(* Logix 5000 AddOnInstructionDefinition export EGU_EGK_IO_Link_Cyclic_Com_1_0_1; software revision 35.00 *)

TYPE PROCESS_DATA_IN :
STRUCT
   B0_00 : BOOL;
   B0_01 : BOOL;
   B0_02 : BOOL;
   B0_03 : BOOL;
   B0_04 : BOOL;
   B0_05 : BOOL;
   B0_06 : BOOL;
   B0_07 : BOOL;
   B0_08 : BOOL;
   B0_09 : BOOL;
   B0_10 : BOOL;
   B0_11 : BOOL;
   B0_12 : BOOL;
   B0_13 : BOOL;
   B0_14 : BOOL;
   B0_15 : BOOL;
   B0_16 : BOOL;
   B0_17 : BOOL;
   B0_18 : BOOL;
   B0_19 : BOOL;
   B0_20 : BOOL;
   B0_21 : BOOL;
   B0_22 : BOOL;
   B0_23 : BOOL;
   B0_24 : BOOL;
   B0_25 : BOOL;
   B0_26 : BOOL;
   B0_27 : BOOL;
   B0_28 : BOOL;
   B0_29 : BOOL;
   B0_30 : BOOL;
   B0_31 : BOOL;
   DINT_1 : DINT;
   DINT_2 : DINT;
   SINT_3_0 : SINT;
   SINT_3_1 : SINT;
   SINT_3_2 : SINT;
   SINT_3_3 : SINT;
END_STRUCT
END_TYPE

TYPE PROCESS_DATA_OUT :
STRUCT
   DINT_0 : DINT;
   DINT_1 : DINT;
   DINT_2 : DINT;
   DINT_3 : DINT;
END_STRUCT
END_TYPE

ADD_ON_INSTRUCTION EGU_EGK_IO_Link_Cyclic_Com_1_0_1   (* revision 1.0 1, ExecutePrescan, ExecuteEnableInFalse *)
// FUNCTION_BLOCK FB_SFP_EGU/EGK Allen Breadley
// TITLE = 'EGU_EGK_Cyclic_Communication'
// VERSION : '1.0.1'
// AUTHOR  : 'SCHUNK'
// NAME    : 'EGU_EGK_Cyclic_Communication'
// FAMILY  : 'SCHUNK'
// Used Products : EGU / EGK
// Projekt Nr.:
// =============================================================================
//  Schunk GmbH&Co.KG
//  (c)Copyright (2022) All Rights Reserved
// -----------------------------------------------------------------------------
//  Library:       Schunk
//  Tested with:   V35.00.00
VAR_INPUT
   b_in_RELEASE_FUNCTION_BLOCK : BOOL; {access Read Only, visible}
   b_in_00_FAST_STOP : BOOL; {access Read Only, visible}
   b_in_01_STOP : BOOL; {access Read Only, visible}
   b_in_02_ACKNOLEDGE : BOOL; {access Read Only, visible}
   b_in_03_PREPARE_FOR_SHUTDOWN : BOOL; {access Read Only, visible}
   b_in_04_SOFTRESET : BOOL; {access Read Only, visible}
   b_in_05_RELEASE_FOR_MANUAL_MOVEMENT : BOOL; {access Read Only, visible}
   b_in_06_REPEAT_COMMAND_TOGGLE : BOOL; {access Read Only, visible}
   b_in_07_GRIP_DIRECTION : BOOL; {access Read Only, visible}
   b_in_08_JOG_MODE_NEGATIVE : BOOL; {access Read Only, visible}
   b_in_09_JOG_MODE_POSITIVE : BOOL; {access Read Only, visible}
   b_in_11_RELEASE_WORKPIECE : BOOL; {access Read Only, visible}
   b_in_12_GRIP_WORKPIECE : BOOL; {access Read Only, visible}
   b_in_13_MOVE_TO_ABSOLUTE_POSITION : BOOL; {access Read Only, visible}
   b_in_14_MOVE_TO_RELATIVE_POSITION : BOOL; {access Read Only, visible}
   b_in_16_GRIP_WORKPIECE_AT_EXPECTED_POS : BOOL; {access Read Only, visible}
   b_in_30_BRAKE_TEST : BOOL; {access Read Only, visible}
   b_in_31_ACTIVATE_GRIP_FORCE_AND_POS_MA : BOOL; {access Read Only, visible}
   di_in_POSITION : DINT; {access Read Only, visible}
   di_in_VELOCITY : DINT; {access Read Only, visible}
   di_in_GRIPPING_FORCE : DINT; {access Read Only, visible}
END_VAR
VAR_OUTPUT
   b_out_00_READY_FOR_OPERATION : BOOL; {visible}
   b_out_01_CONTOL_AUTHORITY_FIELDBUS : BOOL; {visible}
   b_out_02_READY_FOR_SHUTDOWN : BOOL; {visible}
   b_out_03_NOT_FEASIBLE : BOOL; {visible}
   b_out_04_COMMAND_SUCCESSFULLY_PROCESSED : BOOL; {visible}
   b_out_05_COMMAND_RECEIVED_TOGGLE : BOOL; {visible}
   b_out_06_WARNING : BOOL; {visible}
   b_out_07_ERROR : BOOL; {visible}
   b_out_08_RELEASED_FOR_MANUAL_MOVEMENT : BOOL; {visible}
   b_out_09_SOFTWARE_LIMIT_REACHED : BOOL; {visible}
   b_out_11_NO_WORKPIECE_DETECTED : BOOL; {visible}
   b_out_12_WORKPIECE_GRIPPED : BOOL; {visible}
   b_out_13_POSITION_REACHED : BOOL; {visible}
   b_out_14_WORKPIECE_PRE_GRIP_STARTED : BOOL; {visible}
   b_out_16_WORKPIECE_LOST : BOOL; {visible}
   b_out_17_WRONG_WORKPIECE_DETECTED : BOOL; {visible}
   b_out_31_GRIP_FORCE_AND_POS_MAINTAINANC : BOOL; {visible}
   di_out_ACTUAL_POSITION : DINT; {visible}
   si_out_DIAGNOSIS_ERROR : SINT; {visible}
   si_out_DIAGNOSIS_WARNING : SINT; {visible}
   si_out_DIAGNOSIS_WARNING_CODE : SINT;
END_VAR
VAR_INPUT
   in_PROCESS_DATA_INPUT : DINT; {access Read Only}
END_VAR
VAR_IN_OUT
   in_PROZESS_DATA_IO_Link_Gripper : AB:electronic_grippers_EGU__64AA7FB7:I:0; {required}
   out_PROZESS_DATA_IO_Link_Gripper : AB:electronic_grippers_EGU__7038672F:O:0; {required}
END_VAR
VAR
   stat_Input : PROCESS_DATA_IN; {access None}
   stat_Output : PROCESS_DATA_OUT; {access None}
   si_in_INPUT_DATA_GRIPPER_DW_3_0 : SINT; {access Read Only}
   si_in_INPUT_DATA_GRIPPER_DW_3_1 : SINT; {access Read Only}
   si_in_INPUT_DATA_GRIPPER_DW_3_2 : SINT; {access Read Only}
   si_in_INPUT_DATA_GRIPPER_DW_3_3 : SINT; {access Read Only}
END_VAR

ROUTINE EnableInFalse   (* structured text *)
   //////////////////////////////////////////////////////////////
   //   Copyright (c)  <Company Information>
   //--------------------------------------------------------------
   //   Routine: <Routine Name>
   //       Author: <Developer Name>
   //   Created: <Date>
   //--------------------------------------------------------------
   //   Description:
   //
   //   History:
   //
   /////////////////////////////////////////////////////////////
END_ROUTINE

ROUTINE Logic   (* structured text *)
   
   (*
   FUNCTION_BLOCK FB_SFP_EGU/EGK Allen Breadley
   TITLE = 'EGU_EGK_Cyclic_Communication'
   VERSION : '1.0.1'
   AUTHOR  : 'SCHUNK'
   NAME    : 'EGU_EGK_Cyclic_Communication'
   FAMILY  : 'SCHUNK'
   Used Products : EGU / EGK
   Projekt Nr.:
   =============================================================================
    Schunk GmbH&Co.KG
    (c)Copyright (2022) All Rights Reserved
   -----------------------------------------------------------------------------
    Library:       Schunk
    Tested with:   V35.00.00
                   Schunk FW release 5.x
    Engineering:   Studio 5000 V35.00.00
    Restrictions:  XXX(OB types, etc.)
    Requirements:  (hardware, technological package, memory needed, etc.)
    Functionality: The Funktion Block communicates Cyclic with the Gripper to read and wright Data
   
   *************************************************************************
   Historie
   ####################
   1.0.1
   Bugfix
   	di_out_OUTPUT_DATA_Gripper_DW_2 := di_in_VELOCITY;
   	di_out_OUTPUT_DATA_Gripper_DW_3 := di_in_GRIPPING_FORCE;
   ####################
   1.0.0
   Release Funktion Block
   TagType="Base" DataType="BOOL" Usage="Input" Radix="Binary" Required="false" Visible="true" ExternalAccess="Read Only"
   
   *************************************************************************)
   	(*English
   
       Statement section REGION
   
       *************************************************************************
       The function block is TO read AND transfer cyclic parameters that are changed FOR specific functions in the device
       can be used TO make The application process safer OR faster.
   
       Input parameters:
       ------------------
       b_in_RELEASE_FUNCTION_BLOCK				: Release FOR processing the block
   
       b_in_00_FAST_STOP						: immediate shutdown OF The process currently running in The gripper AND shutdown OF The motor phases
       b_in_01_STOP							: Pausing AND stopping the currently running process.
       b_in_02_ACKNOLEDGE						: Acknowledge fault
       b_in_03_PREPARE_FOR_SHUTDOWN			: Initiate the restoration OF data on The device in preparation FOR switching off OR rebooting
       b_in_04_SOFTRESET						: Warm start OF The device
       b_in_05_RELEASE_FOR_MANUAL_MOVEMENT		: The brake can be released FOR 5 seconds in the "ERROR_FAST_STOP" state
       b_in_06_REPEAT_COMMAND_TOGGLE			: The command that is still pending can, IF it is a repeatable command, be repeated without loss OF Time FOR each positive AND negative change OF this bit
       b_in_07_GRIP_DIRECTION					: determines The gripping direction. FALSE = external gripping (the workpiece is gripped from the outside) / True = internal gripping (the workpiece is gripped from the inside).
   
       b_in_08_JOG_MODE_NEGATIVE				: Simple movement OF The device in negative direction. Function also possible without "REFERENCE".
       b_in_09_JOG_MODE_POSITIVE				: Simple movement OF The device in The positive direction. Function also possible without "REFERENCE".
   
       b_in_11_RELEASE_WORKPIECE				: IF The status is "GRIPPED", the gripper is opened in the opposite direction AND the workpiece is released
       b_in_12_GRIP_WORKPIECE					: the gripper executes a movement that should lead TO gripping a workpiece. Internal speed parameters are used here
       b_in_13_MOVE_TO_ABSOLUTE_POSITION		: the gripper jaws are moved TO The position specified in The cyclic protocol at The specified speed.
       b_in_14_MOVE_TO_RELATIVE_POSITION		: the gripper jaws are moved TO The calculated position with The position specified in The cyclic protocol at The specified speed.
   
       b_in_16_GRIP_WORKPIECE_AT_EXPECTED_POSITION :  the gripper performs a gripping run on a specified workpiece. first a positioning run to the pre-position and then a gripping run to the workpiece.
       b_in_30_BRAKE_TEST						: the gripper activates the brake and energizes the motor
   	b_in_31_ACTIVATE_GRIP_FORCE_AND_POSITION_MAINTENANCE  :  sets the use of gripping force and position maintenance ( False = GPE is not used / True = GPE is activated)
   
       di_in_POSITION							: Entry of the absolute or relative position in µm
       di_in_VELOCITY							: Entry of the speed when positioning gripping mm/sec
       di_in_GRIPPING_FORCE					: Entry of the gripping force is entered in %. Here you can read in the manual which gripping modes should be used. The indication of the gripping force can then be selected accordingly.
   
       di_in_INPUT_DATA_GRIPPER_DW_0			: Input Data DoubleWord 0 of the Gripper
       di_in_INPUT_DATA_GRIPPER_DW_0			: Input Data DoubleWord 1 of the Gripper
       di_in_INPUT_DATA_GRIPPER_DW_0			: Input Data DoubleWord 2 of the Gripper
       di_in_INPUT_DATA_GRIPPER_DW_0			: Input Data DoubleWord 3 of the Gripper
   
       #################
   
       Output parameters:
       ------------------
   
       b_out_00_READY_FOR_OPERATION            : indicates that the gripper is ready FOR operation
       b_out_01_CONTOL_AUTHORITY_FIELDBUS      : indicates whether the fieldbus has control authority over the gripper
       b_out_02_READY_FOR_SHUTDOWN             : signals readiness FOR shutdown OR restart after the request "Prepare for shutdown"
       b_out_03_NOT_FEASIBLE                   : Indicates that the last issued command cannot be executed.
                                               Possible causes are:
                                               - a new command was sent although the command that is still active has NOT yet been processed.
                                               - 2 OR more control commands simultaneously active in the control word
                                               - Parameter data FOR position, speed OR force are outside the permissible limits.
   
       b_out_04_COMMAND_SUCCESSFULLY_PROCESSED : indicates that the last executable command was successfully processed.
       b_out_05_COMMAND_RECEIVED_TOGGLE        : indicates that a command was sent TO The gripper via The bus. the command does NOT have TO be processed OR started at the time it is displayed.
       b_out_06_WARNING                        : signals a warning in the gripper, e.g. temperature warning
       b_out_07_ERROR                          : signals a fault in the gripper, e.g. rapid stop
       b_out_08_RELEASD_FOR_MANUAL_MOVEMENT    : Signals that the brake is released IF a brake is installed in the gripper.
       b_out_09_SOFTWARELIMIT_REACHED          : indicates that the gripper has reached a software limit
   
       b_out_11_NO_WORKPIECE_DETECTED          : indicates that no workpiece was detected
       b_out_12_WORKPIECE_GRIPPED              : signals that a workpiece has been gripped
       b_out_13_POSITION_REACHED               : signals that the relative OR absolute position has been approached
       b_out_14_WORKPIECE_PRE_GRIPPED_STARTED  : indicates that the gripper has started the pre-gripping function
       b_out_16_WORKPIECE_LOST                 : signals that the gripped workpiece was lost
       b_out_17_WRONG_WORKPIECE_DETECTED       : signals that a wrong workpiece was detected
       b_out_31_GRIP_FORCE_AND_POSITION_MAINTAINANCE_ACTIVATED : signals that GPE is active
   
       di_out_ACTUAL_POSITION                  : the current position OF The gripper is returned here
       i_out_DIAGNOSE_WARNUNG                  : Output of the gripper's warning code
       i_out_DIAGNOSE_ERROR                    : Output of the error code of the gripper
   
       di_out_OUTPUT_DATA_Gripper_DW_0			: Output Data DoubleWord 0 of the Gripper
       di_out_OUTPUT_DATA_Gripper_DW_1			: Output Data DoubleWord 1 of the Gripper
       di_out_OUTPUT_DATA_Gripper_DW_2			: Output Data DoubleWord 2 of the Gripper
       di_out_OUTPUT_DATA_Gripper_DW_3			: Output Data DoubleWord 3 of the Gripper
   
       *************************************************************************)
   
   
   (*************************************************************************
       German
   
   	Der Baustein soll Zyklische Parameter einlesen und übertragen, welche für bestimmte Funktionen im Gerät geändert
       werden können um den Applikationsprozess sicherer oder schneller zu machen.
   
       Eingangsparameter:
       ------------------
   
       b_RELEASE_FUNCTION_BLOCK            : Freigabe zur Bearbeitung des Bausteins (True = Freigabe zur Bearbeitung)
   
       b_00_FAST_STOP                      : sofortiges Abschalten des aktuell im Greifer laufenden Prozesses und abschalten der Motorphasen
       b_01_STOP                           : Anhalten und Stoppen des Aktuell laufenden Prozesses.
       b_02_ACKNOLEDGE                     : Störung Quittieren
       b_03_PREPARE_FOR_SHUTDOWN           : Anstoßen der Rückspeicherung von Daten auf dem Grät un Vorbereitung zum Ausschalten oder Reboot
       b_04_SOFTRESET                      : Warmstart des Gerätes
       b_05_RELEASE_FOR_MANUAL_MOVEMENT    : Lösen der Bremse für 5 Sekunden im Zustand "ERROR_FAST_STOP" möglich
       b_06_REPEAT_COMMAND_TOGGLE          : Das Noch anstehende Kommando kann, sofern es ein wiederholbares Kommando ist, ohne zeitverlust bei jedem positiven und negativen wechsel dieses Bits wiederholt werden
       b_07_GRIP_DIRECTION                 : legt die Greifrichtung fest. FALSE = Ausengreifen (Das Werkstück wird von ausen gegriffen) / True = Innengreifen (Das Werkstück wird von innen gegriffen).
   
       b_08_JOG_MODE_NEGATIVE              : einfaches Verfahren des Gerätes in negative Richtung. Funktion auch ohne Referenz möglich.
       b_09_JOG_MODE_POSITIVE              : einfaches Verfahren des Gerätes in positive Richtung. Funktion auch ohne Referenz möglich.
   
       b_11_RELEASE_WORKPIECE              : Bei Status "GRIPPED" wird der Greifer in die entgegegesetzte Richtung geöffnet und das Werkstück freigegeben
       b_12_GRIP_WORKPIECE                 : der Greifer führt eine Bewegung aus, welche zum greifen eines Werkstückes führen soll. Hierbei werden interne Geschwindigkeitsparameter genommen
       b_13_MOVE_TO_ABSOLUTE_POSITION      : Die Greiferbacken werden auf die im Zyklischen Protokoll vorgegebene Position mit der vorgegebenen Geschwindigkeit gefahren.
       b_14_MOVE_TO_RELATIVE_POSITION      : Die Greiferbacken werden auf die errechnete Position mit der im Zyklischen Protokoll vorgegebene Position mit der vorgegebenen Geschwindigkeit gefahren.
   
       b_16_GRIP_WORKPIECE_AT_EXPECTED_POSITION            : Der Greifer führt eine Greiffahrt auf ein vorgegebenes Werkstück aus. Hierbei wird zuerst eine Positionsfahrt auf die Vorposition um dann mit einer Greiffahrt auf das Werkstück zu fahren.
       b_in_30_BRAKE_TEST						: der Greifer aktiviert die Bremse und bestromt den Motor
   	b_31_ACTIVATE_GRIP_FORCE_AND_POSITION_MAINTENANCE   : legt die Verwendung der Greifkaft und Positionserhaltung fest ( False = GPE wird nicht verwendet / True = GPE wird aktiviert)
   
       di_POSITION                         : Eintrag der Absoluten oder Relativen Possition in µm
       di_VELOCITY                         : Eintrag der Geschwindigkeit beim Possitioniern Greifen mm/Sec
       di_GRIPPING_FORCE                   : Eintrag der Greifkraft wird in % eingetragen. Hier ist im Handbuch nachzulesen welcher Greifmodi verwendet werden soll. Entsprechend kann dann die angabe der Greifkraft gewählt werden.
   
       INPUT_DATA_GRIPPER_DW_0		:	Eingangsdaten Doppelwort 0 des Greifers
       INPUT_DATA_GRIPPER_DW_0		:	Eingangsdaten Doppelwort 1 des Greifers
       INPUT_DATA_GRIPPER_DW_0		:	Eingangsdaten Doppelwort 2 des Greifers
       INPUT_DATA_GRIPPER_DW_0		:	Eingangsdaten Doppelwort 3 des Greifers
   
       ##################
   
   
       Ausgangsparameter:
       ------------------
   
       b_out_00_READY_FOR_OPPERATION           : zeigt die Betriebsbereitschaft des Greifers an
       b_out_01_CONTOL_AUTHORITY_FIELDBUS      : zeigt an, ob der Feldbus die Steuerhoheit über den Greifer hat
       b_out_02_READY_FOR_SHUTDOWN             : signalisiert die Bereitschaft zum Abschalten bzw Neustarten nach der Anforderung "Prepare for shutdown"
       b_out_03_NOT_FEASIBLE                   : Zeigt an, das der zuletzt abgesetzte Befehl nicht ausgeführt werden kann.
                                               Mögliche Ursachen sind:
                                               - ein neuer Befehl wurde abgesetzt, obwohl der noch aktive Befehl noch nicht abgearbeitet wurde.
                                               - 2 oder mehr Steuerbefehle gleichzeitig aktiv im Steuerwort
                                               - Parameterdaten von Position, Geschwindigkeit oder Kraft liegen auserhalb der Zulässigen grenzen.
   
       b_out_04_COMMAND_SUCCESSFULLY_PROCESSED : zeigt das erfolgreiche Abarbeiten des letzten ausführbaren Befehls an.
       b_out_05_COMMAND_RECEIVED_TOGGLE        : Zeigt an, das ein Befehl über den Bus an den Greufer gesendet wurde. Zum Zeitpunkt der Anzeige muß der Befehl noch nicht abgearbeitet oder gestartet sein.
       b_out_06_WARNING                        : signalisiert eine Warnung im Greifer, z.B. Temperaturwarnung
       b_out_07_ERROR                          : signalisiert eine Störung im Greifer, z.B. Schnellstop
       b_out_08_RELEASD_FOR_MANUAL_MOVEMENT    : Signalisiert, dass die Bremse geöffnet ist, sofern eine Bremse im Greifer verbaut ist.
       b_out_09_SOFTWARELIMIT_REACHED          : signalisiert, das der Greifer eine Softwarelimit angefahren hat
       b_out_10_REFERENCED                     : signalisiert, das der Greifer referenziert ist
       b_out_11_NO_WORKPIECE_DETECTED          : signalisiert, dass kein Werkstück erkannt wurde
       b_out_12_WORKPIECE_GRIPPED              : signalisiert, dass ein Werkstück gegriffen wurde
       b_out_13_POSITION_REACHED               : signalisiert, dass die relative oder absolute Possition angefahren wurde
       b_out_14_WORKPIECE_PRE_GRIPPED_STARTED  : signalisiert, dass der Greifer die Pre Gripping Funktion angestoßen hat
       b_out_16_WORKPIECE_LOST                 : signalisiert, dass das gegriffene Werkstück verloren ging
       b_out_17_WRONG_WORKPIECE_DETECTED       : signalisiert, das ein falsches Werkstück erkannt wurde
       b_out_31_GRIP_FORCE_AND_POSITION_MAINTAINANCE_ACTIVATED :   Signalisiert, dass GPE aktiev ist
   
       di_out_ACTUAL_POSITION                  : hier wird die aktuelle Possition des Greifers zurückgegeben
       i_out_DIAGNOSE_WARNUNG                  : Ausgabe des Warnungscodes des Greifers
       i_out_DIAGNOSE_ERROR                    : Ausgabe des Störungscodes des Greifers
   
       di_out_OUTPUT_DATA_Gripper_DW_0		: Output Data DoubleWord 0 of the Gripper
       di_out_OUTPUT_DATA_Gripper_DW_1		: Output Data DoubleWord 1 of the Gripper
       di_out_OUTPUT_DATA_Gripper_DW_2		: Output Data DoubleWord 2 of the Gripper
       di_out_OUTPUT_DATA_Gripper_DW_3		: Output Data DoubleWord 3 of the Gripper
   *************************************************************************)
   
   
       IF NOT b_in_RELEASE_FUNCTION_BLOCK
   
       THEN
   
   	out_PROZESS_DATA_IO_Link_Gripper.fast_stop 									:= 0;
   	out_PROZESS_DATA_IO_Link_Gripper.stop 										:= 0;
   	out_PROZESS_DATA_IO_Link_Gripper.acknowledge 								:= 0;
   	out_PROZESS_DATA_IO_Link_Gripper.prepare_for_shutdown 						:= 0;
   	out_PROZESS_DATA_IO_Link_Gripper.softreset									:= 0;
   	out_PROZESS_DATA_IO_Link_Gripper.release_for_manual_movement				:= 0;
   	// out_PROZESS_DATA_IO_Link_Gripper.repeat_command_toggle						:= 0;
   	// out_PROZESS_DATA_IO_Link_Gripper.grip_direction								:= 0;
   	out_PROZESS_DATA_IO_Link_Gripper.jog_mode_negative							:= 0;
   	out_PROZESS_DATA_IO_Link_Gripper.jog_mode_positive							:= 0;
   	out_PROZESS_DATA_IO_Link_Gripper.reserved_10								:= 0;
   	out_PROZESS_DATA_IO_Link_Gripper.release_workpiece							:= 0;
   	out_PROZESS_DATA_IO_Link_Gripper.grip_workpiece								:= 0;
   	out_PROZESS_DATA_IO_Link_Gripper.move_to_absolute_position					:= 0;
   	out_PROZESS_DATA_IO_Link_Gripper.move_to_absolute_position					:= 0;
   	out_PROZESS_DATA_IO_Link_Gripper.reserved_15								:= 0;
   	out_PROZESS_DATA_IO_Link_Gripper.grip_workpiece_at_expected_position		:= 0;
   	out_PROZESS_DATA_IO_Link_Gripper.reserved_17								:= 0;
   	out_PROZESS_DATA_IO_Link_Gripper.reserved_18								:= 0;
   	out_PROZESS_DATA_IO_Link_Gripper.reserved_19								:= 0;
   	out_PROZESS_DATA_IO_Link_Gripper.reserved_20								:= 0;
   	out_PROZESS_DATA_IO_Link_Gripper.reserved_21								:= 0;
   	out_PROZESS_DATA_IO_Link_Gripper.reserved_22								:= 0;
   	out_PROZESS_DATA_IO_Link_Gripper.reserved_23								:= 0;
   	out_PROZESS_DATA_IO_Link_Gripper.reserved_24								:= 0;
   	out_PROZESS_DATA_IO_Link_Gripper.reserved_25								:= 0;
   	out_PROZESS_DATA_IO_Link_Gripper.reserved_26								:= 0;
   	out_PROZESS_DATA_IO_Link_Gripper.reserved_27								:= 0;
   	out_PROZESS_DATA_IO_Link_Gripper.reserved_28								:= 0;
   	out_PROZESS_DATA_IO_Link_Gripper.reserved_29								:= 0;
   	out_PROZESS_DATA_IO_Link_Gripper.brake_test									:= 0;
   	out_PROZESS_DATA_IO_Link_Gripper.use_grip_force_and_position_maintenance	:= 0;
   
   	out_PROZESS_DATA_IO_Link_Gripper.positioning_parameter						:= 0;
   	out_PROZESS_DATA_IO_Link_Gripper.velocity_parameter							:= 0;
   	out_PROZESS_DATA_IO_Link_Gripper.gripping_force_parameter					:= 0;
   
   		TND( ); // Temp End
   
       END_IF;
   
   	// Read the Cyclic Date
   	// Einlesen der Zyklischen Daten
   
   		//stat_Input.DINT_0	:= udt_in_PROZESS_DATA_IN.DINT_0;
   		//stat_Input.DINT_1	:= in_PROZESS_DATA_IO_Link_Gripper.DINT_1;
   		//stat_Input.DINT_2	:= in_PROZESS_DATA_IO_Link_Gripper.DINT_2;
   
   		//stat_Input.SINT_3_0	:= in_PROZESS_DATA_IO_Link_Gripper.SINT_3_0;
   		//stat_Input.SINT_3_1 := in_PROZESS_DATA_IO_Link_Gripper.SINT_3_1;
   		//stat_Input.SINT_3_2	:= in_PROZESS_DATA_IO_Link_Gripper.SINT_3_2;
   		//stat_Input.SINT_3_3	:= in_PROZESS_DATA_IO_Link_Gripper.SINT_3_3;
   
       // Enter the input data in the instance DB and assign them to the status displays
       // Eingangsdaten in den Instanz DB eintragen und den Statusanzeigen zuweisen
   
   	b_out_00_READY_FOR_OPERATION 			:= in_PROZESS_DATA_IO_Link_Gripper.ready_for_operation;
   	b_out_01_CONTOL_AUTHORITY_FIELDBUS 		:= in_PROZESS_DATA_IO_Link_Gripper.ctrl_authority_fieldbus;
   	b_out_02_READY_FOR_SHUTDOWN 			:= in_PROZESS_DATA_IO_Link_Gripper.ready_for_shutdown;
   	b_out_03_NOT_FEASIBLE 					:= in_PROZESS_DATA_IO_Link_Gripper.not_feasible;
   	b_out_04_COMMAND_SUCCESSFULLY_PROCESSED := in_PROZESS_DATA_IO_Link_Gripper.command_successfully_processed;
   	b_out_05_COMMAND_RECEIVED_TOGGLE 		:= in_PROZESS_DATA_IO_Link_Gripper.command_received_toggle;
   	b_out_06_WARNING 						:= in_PROZESS_DATA_IO_Link_Gripper.warning;
   	b_out_07_ERROR 							:= in_PROZESS_DATA_IO_Link_Gripper.error;
   	b_out_08_RELEASED_FOR_MANUAL_MOVEMENT 	:= in_PROZESS_DATA_IO_Link_Gripper.released_for_manual_movement;
   	b_out_09_SOFTWARE_LIMIT_REACHED 		:= in_PROZESS_DATA_IO_Link_Gripper.software_limit_reached;
   	b_out_11_NO_WORKPIECE_DETECTED 			:= in_PROZESS_DATA_IO_Link_Gripper.no_workpiece_detected;
   	b_out_12_WORKPIECE_GRIPPED 				:= in_PROZESS_DATA_IO_Link_Gripper.workpiece_gripped;
   	b_out_13_POSITION_REACHED 				:= in_PROZESS_DATA_IO_Link_Gripper.position_reached;
   	b_out_14_WORKPIECE_PRE_GRIP_STARTED 	:= in_PROZESS_DATA_IO_Link_Gripper.workpiece_pre_grip_started;
   	b_out_16_WORKPIECE_LOST 				:= in_PROZESS_DATA_IO_Link_Gripper.workpiece_lost;
   	b_out_17_WRONG_WORKPIECE_DETECTED 		:= in_PROZESS_DATA_IO_Link_Gripper.wrong_workpiece_gripped;
   	b_out_31_GRIP_FORCE_AND_POS_MAINTAINANC := in_PROZESS_DATA_IO_Link_Gripper.grip_force_and_position_maintenance_used;
   
   
   	di_out_ACTUAL_POSITION 					:= in_PROZESS_DATA_IO_Link_Gripper.actual_Position;
   	si_out_DIAGNOSIS_ERROR 					:= in_PROZESS_DATA_IO_Link_Gripper.error_code;
   
   	si_out_DIAGNOSIS_WARNING 				:= in_PROZESS_DATA_IO_Link_Gripper.warning_code;
   	si_out_DIAGNOSIS_WARNING_CODE 			:= in_PROZESS_DATA_IO_Link_Gripper.additional_warning_code;
   
   
       // Allocation of output data for the periphery
       // Zuweisung der Ausgangsdaten für die Peripher
   
   	out_PROZESS_DATA_IO_Link_Gripper.fast_stop 									:= b_in_00_FAST_STOP;
   	out_PROZESS_DATA_IO_Link_Gripper.stop 										:= b_in_01_STOP;
   	out_PROZESS_DATA_IO_Link_Gripper.acknowledge 								:= b_in_02_ACKNOLEDGE;
   	out_PROZESS_DATA_IO_Link_Gripper.prepare_for_shutdown 						:= b_in_03_PREPARE_FOR_SHUTDOWN;
   	out_PROZESS_DATA_IO_Link_Gripper.softreset									:= b_in_04_SOFTRESET;
   	out_PROZESS_DATA_IO_Link_Gripper.release_for_manual_movement				:= b_in_05_RELEASE_FOR_MANUAL_MOVEMENT;
   	out_PROZESS_DATA_IO_Link_Gripper.repeat_command_toggle						:= b_in_06_REPEAT_COMMAND_TOGGLE;
   	out_PROZESS_DATA_IO_Link_Gripper.grip_direction								:= b_in_07_GRIP_DIRECTION;
   	out_PROZESS_DATA_IO_Link_Gripper.jog_mode_negative							:= b_in_08_JOG_MODE_NEGATIVE;
   	out_PROZESS_DATA_IO_Link_Gripper.jog_mode_positive							:= b_in_09_JOG_MODE_POSITIVE;
   	out_PROZESS_DATA_IO_Link_Gripper.reserved_10								:= 0;
   	out_PROZESS_DATA_IO_Link_Gripper.release_workpiece							:= b_in_11_RELEASE_WORKPIECE;
   	out_PROZESS_DATA_IO_Link_Gripper.grip_workpiece								:= b_in_12_GRIP_WORKPIECE;
   	out_PROZESS_DATA_IO_Link_Gripper.move_to_absolute_position					:= b_in_13_MOVE_TO_ABSOLUTE_POSITION;
   	out_PROZESS_DATA_IO_Link_Gripper.move_to_absolute_position					:= b_in_14_MOVE_TO_RELATIVE_POSITION;
   	out_PROZESS_DATA_IO_Link_Gripper.reserved_15								:= 0;
   	out_PROZESS_DATA_IO_Link_Gripper.grip_workpiece_at_expected_position		:= b_in_16_GRIP_WORKPIECE_AT_EXPECTED_POS;
   	out_PROZESS_DATA_IO_Link_Gripper.reserved_17								:= 0;
   	out_PROZESS_DATA_IO_Link_Gripper.reserved_18								:= 0;
   	out_PROZESS_DATA_IO_Link_Gripper.reserved_19								:= 0;
   	out_PROZESS_DATA_IO_Link_Gripper.reserved_20								:= 0;
   	out_PROZESS_DATA_IO_Link_Gripper.reserved_21								:= 0;
   	out_PROZESS_DATA_IO_Link_Gripper.reserved_22								:= 0;
   	out_PROZESS_DATA_IO_Link_Gripper.reserved_23								:= 0;
   	out_PROZESS_DATA_IO_Link_Gripper.reserved_24								:= 0;
   	out_PROZESS_DATA_IO_Link_Gripper.reserved_25								:= 0;
   	out_PROZESS_DATA_IO_Link_Gripper.reserved_26								:= 0;
   	out_PROZESS_DATA_IO_Link_Gripper.reserved_27								:= 0;
   	out_PROZESS_DATA_IO_Link_Gripper.reserved_28								:= 0;
   	out_PROZESS_DATA_IO_Link_Gripper.reserved_29								:= 0;
   	out_PROZESS_DATA_IO_Link_Gripper.brake_test									:= b_in_30_BRAKE_TEST;
   	out_PROZESS_DATA_IO_Link_Gripper.use_grip_force_and_position_maintenance	:= b_in_31_ACTIVATE_GRIP_FORCE_AND_POS_MA;
   
   
   	out_PROZESS_DATA_IO_Link_Gripper.positioning_parameter						:= di_in_POSITION;
   	out_PROZESS_DATA_IO_Link_Gripper.velocity_parameter							:= di_in_VELOCITY;
   	out_PROZESS_DATA_IO_Link_Gripper.gripping_force_parameter					:= di_in_GRIPPING_FORCE;
   
END_ROUTINE

ROUTINE Postscan   (* structured text *)
   //////////////////////////////////////////////////////////////
   //   Copyright (c)  <Company Information>
   //--------------------------------------------------------------
   //   Routine: <Routine Name>
   //       Author: <Developer Name>
   //   Created: <Date>
   //--------------------------------------------------------------
   //   Description:
   //
   //   History:
   //
   /////////////////////////////////////////////////////////////
END_ROUTINE

ROUTINE Prescan   (* structured text *)
   //////////////////////////////////////////////////////////////
   //   Copyright (c)  <Company Information>
   //--------------------------------------------------------------
   //   Routine: <Routine Name>
   //       Author: <Developer Name>
   //   Created: <Date>
   //--------------------------------------------------------------
   //   Description:
   //
   //   History:
   //
   /////////////////////////////////////////////////////////////
END_ROUTINE
END_ADD_ON_INSTRUCTION
